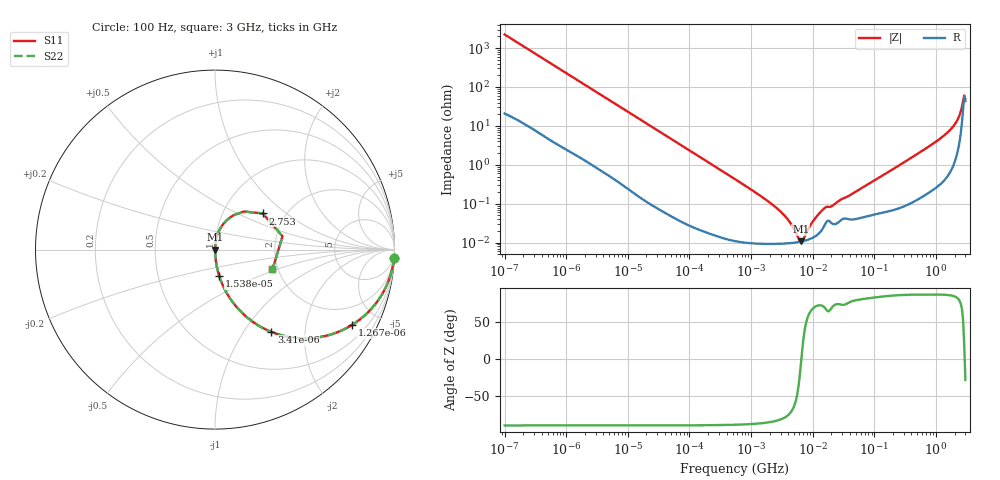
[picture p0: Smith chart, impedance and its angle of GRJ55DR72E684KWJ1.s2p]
!Murata Part Number: GRJ55DR72E684KWJ1
!These Parameters are Measured in Series Mode Connection
!Data Generated on Jun 19, 2026
!  o--ll--o
!Port1  Port2
!  o------o
!Operation Temp=25[degC], DC Bias Voltage=0[V]
!Freq. Start=100[Hz] Stop=3[GHz] 401[Steps]
# Hz S RI R 50
!Freq.(Hz) S11(Real) S11(Imag) S21(Real) S21(Imag) S12(Real) S12(Imag) S22(Real) S22(Imag)
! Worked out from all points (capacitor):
!   401 points, 100 Hz to 3 GHz, reference 50 ohm
!   read as one part in series: C = 708 nF near 109 Hz
!   lowest |Z| = 10.8 mohm at 6.369 MHz (marker M1)
!   series resonance near 6.543 MHz, so ESL is about 840 pH
!   S11 on the Smith chart (normalised r, x): 100 Hz: 1, -45; 1.267 kHz: 1.04, -3.60; 3.41 kHz: 1.02, -1.35; 15.38 kHz: 1.00, -0.30; 2.753 GHz: 1.53, +0.70; 3 GHz: 1.87, -0.47
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100  0.9976 -0.0445  0.00239 0.0445  0.00239 0.0445  0.9976 -0.0445
492  0.9532 -0.206  0.0468 0.206  0.0468 0.206  0.9532 -0.206
1267  0.7621 -0.4203  0.2379 0.4203  0.2379 0.4203  0.7621 -0.4203
1788  0.6198 -0.4798  0.3802 0.4798  0.3802 0.4798  0.6198 -0.4798
3410  0.3147 -0.4588  0.6853 0.4588  0.6853 0.4588  0.3147 -0.4588
6504  0.1148 -0.3134  0.8852 0.3134  0.8852 0.3134  0.1148 -0.3134
15384  0.0237 -0.1473  0.9763 0.1473  0.9763 0.1473  0.0237 -0.1473
31977  0.006 -0.0725  0.994 0.0725  0.994 0.0725  0.006 -0.0725
547723  0.000128 -0.00429  0.9999 0.00429  0.9999 0.00429  0.000128 -0.00429
2934810  9.43e-05 -0.000646  0.9999 0.000646  0.9999 0.000646  9.43e-05 -0.000646
4141163  9.7e-05 -0.000344  0.9999 0.000344  0.9999 0.000344  9.7e-05 -0.000344
6368694  0.000106 -1.95e-05  0.9999 1.95e-05  0.9999 1.95e-05  0.000106 -1.95e-05
7246509  0.000111 7.48e-05  0.9999 -7.48e-05  0.9999 -7.48e-05  0.000111 7.48e-05
9794414  0.000132 0.000305  0.9999 -0.000305  0.9999 -0.000305  0.000132 0.000305
1.572531e7  0.000289 0.000732  0.9997 -0.000732  0.9997 -0.000732  0.000289 0.000732
1.751444e8  0.000692 0.00676  0.9993 -0.00676  0.9993 -0.00676  0.000692 0.00676
1.443257e9  0.0082 0.0612  0.9918 -0.0612  0.9918 -0.0612  0.0082 0.0612
1.950712e9  0.0203 0.0988  0.9797 -0.0988  0.9797 -0.0988  0.0203 0.0988
2.317205e9  0.0501 0.1476  0.9499 -0.1476  0.9499 -0.1476  0.0501 0.1476
2.525516e9  0.1017 0.1908  0.8982 -0.1908  0.8982 -0.1908  0.1017 0.1908
2.752553e9  0.2659 0.2014  0.7341 -0.2014  0.7341 -0.2014  0.2659 0.2014
3e9  0.32 -0.1108  0.68 0.1108  0.68 0.1108  0.32 -0.1108
